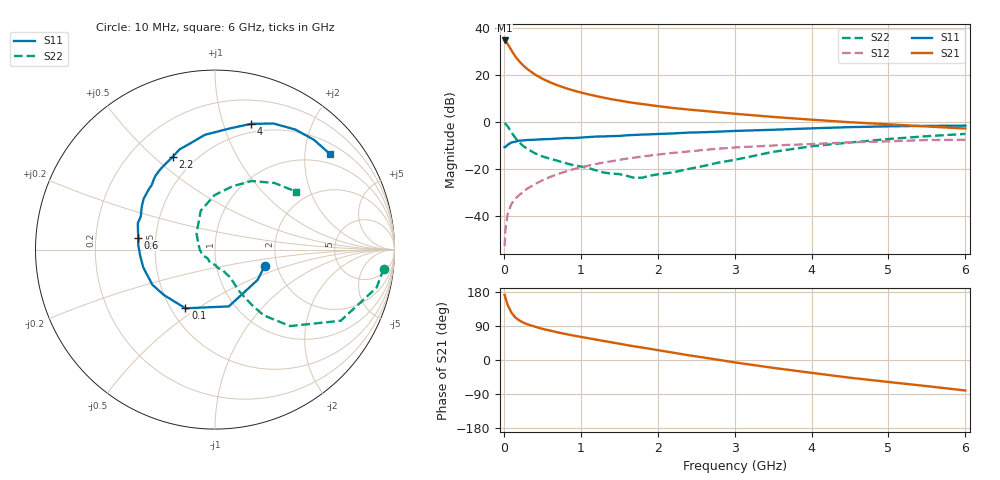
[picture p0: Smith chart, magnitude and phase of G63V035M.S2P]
! SIEMENS Small Signal Semiconductors
! BFG193
! Si NPN RF Bipolar Junction Transistor in SOT223
! VCE = 3 V  IC = 35 mA
! Common Emitter S-Parameters:  August  1996
# GHz  S  MA  R  50
!  f  S11  S21  S12  S22
! GHz  MAG  ANG  MAG  ANG  MAG  ANG  MAG  ANG
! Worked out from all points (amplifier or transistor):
!   36 points, 10 MHz to 6 GHz, reference 50 ohm
!   highest |S21| = 34.6 dB at 10 MHz (marker M1)
!   |S21| within 3 dB of that: start of sweep to 76.86 MHz
!   unconditionally stable (mu >= 1): 491.5 MHz to 2.411 GHz
!   at 250 MHz: K = 0.87, MSG = 26.8 dB, |S12| = -29.7 dB
!   at 1.4 GHz: K = 1.05, MAG = 11.9 dB, |S12| = -16.7 dB
!   at 6 GHz: K = 0.90, MSG = 2.4 dB, |S12| = -7.6 dB
!   S11 on the Smith chart (normalised r, x): 10 MHz: 1.73, -0.34; 100 MHz: 0.59, -0.45; 600 MHz: 0.40, +0.07; 2.2 GHz: 0.38, +0.58; 4 GHz: 0.41, +1.24; 6 GHz: 0.74, +2.58
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0.01  0.2915 -17.8  53.58 171.6  0.0023 85.3  0.9459 -6.4
0.02  0.2915 -35.3  52.07 164.7  0.005 80.6  0.9251 -13.2
0.05  0.3257 -76.3  44.91 144.7  0.0112 73.0  0.8048 -29.5
0.1  0.3661 -116.7  32.8 124.9  0.0183 64.8  0.5974 -45.5
0.15  0.3809 -138.3  24.42 112.0  0.0234 63.5  0.4553 -53.5
0.2  0.4 -150.7  19.39 104.7  0.0279 64.2  0.3706 -56.3
0.25  0.4033 -159.4  15.88 99.1  0.0329 64.6  0.3086 -58.3
0.3  0.412 -166.1  13.45 94.7  0.0378 65.8  0.2715 -59.7
0.4  0.4183 -175.3  10.26 88.3  0.0474 65.9  0.2173 -60.5
0.5  0.4279 176.8  8.253 82.3  0.0574 65.6  0.185 -60.9
0.6  0.4325 171.1  6.938 77.6  0.0678 65.3  0.1655 -62.4
0.8  0.4545 161.1  5.23 68.8  0.088 62.5  0.1334 -67.5
1.1  0.4763 148.5  3.841 57.5  0.1179 57.6  0.1045 -80.2
1.3  0.4919 141.5  3.261 50.1  0.1376 53.6  0.0841 -90.9
1.6  0.5194 131.0  2.658 39.3  0.1661 46.9  0.0717 -117.3
2.2  0.5691 114.3  1.975 19.4  0.22 33.6  0.0847 -179.7
2.8  0.622 99.3  1.594 0.1  0.2707 19.6  0.1377 138.5
3.5  0.6807 82.9  1.275 -20.7  0.3153 2.4  0.2313 110.0
4  0.7296 73.9  1.115 -33.9  0.3387 -7.4  0.3038 90.4
4.5  0.7749 65.0  0.983 -46.8  0.3686 -17.5  0.3655 74.7
5.5  0.8235 48.0  0.8 -69.0  0.4123 -40.7  0.4973 48.3
6  0.8328 39.8  0.724 -80.5  0.417 -54.0  0.5555 35.6
